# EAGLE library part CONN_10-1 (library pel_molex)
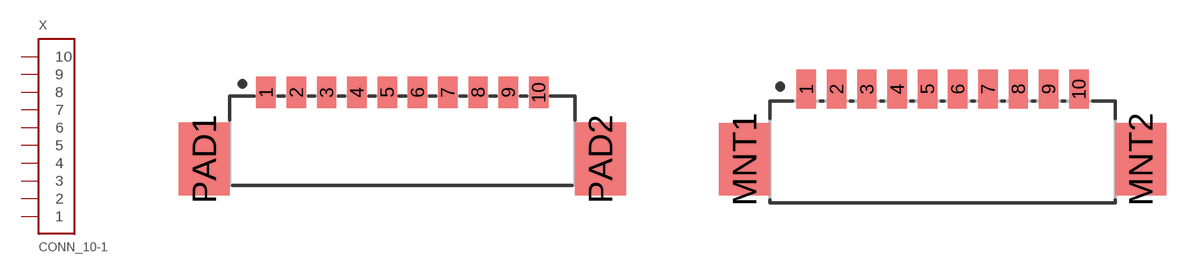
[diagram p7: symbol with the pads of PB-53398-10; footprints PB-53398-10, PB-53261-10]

Designator prefix X

## CONN_10-1-53398  [PB-53398-10]
1  1
2  2
3  3
4  4
5  5
6  6
7  7
8  8
9  9
10  10

## CONN_10-1-53261  [PB-53261-10]
Pads as for PB-53398-10

## CONN_10-1-53047  [PB-53047-10]
Pads as for PB-53398-10

## Footprint PB-53398-10 (pad centres in mm)
smd 0.8 x 1.3: 1 -5.625,1.25; 2 -4.375,1.25; 3 -3.125,1.25; 4 -1.875,1.25; 5 -0.625,1.25; 6 0.625,1.25; 7 1.875,1.25; 8 3.125,1.25; 9 4.375,1.25; 10 5.625,1.25
smd 2.1 x 3: PAD1 -8.175,-1.5; PAD2 8.175,-1.5

## Footprint PB-53261-10 (pad centres in mm)
smd 0.8 x 1.6: 1 -5.625,1.1; 2 -4.375,1.1; 3 -3.125,1.1; 4 -1.875,1.1; 5 -0.625,1.1; 6 0.625,1.1; 7 1.875,1.1; 8 3.125,1.1; 9 4.375,1.1; 10 5.625,1.1
smd 2.1 x 3: MNT1 -8.175,-1.8; MNT2 8.175,-1.8

## Footprint PB-53047-10 (pad centres in mm)
drill 0.5: 1 -5.625,0; 2 -4.375,0; 3 -3.125,0; 4 -1.875,0; 5 -0.625,0; 6 0.625,0; 7 1.875,0; 8 3.125,0; 9 4.375,0; 10 5.625,0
